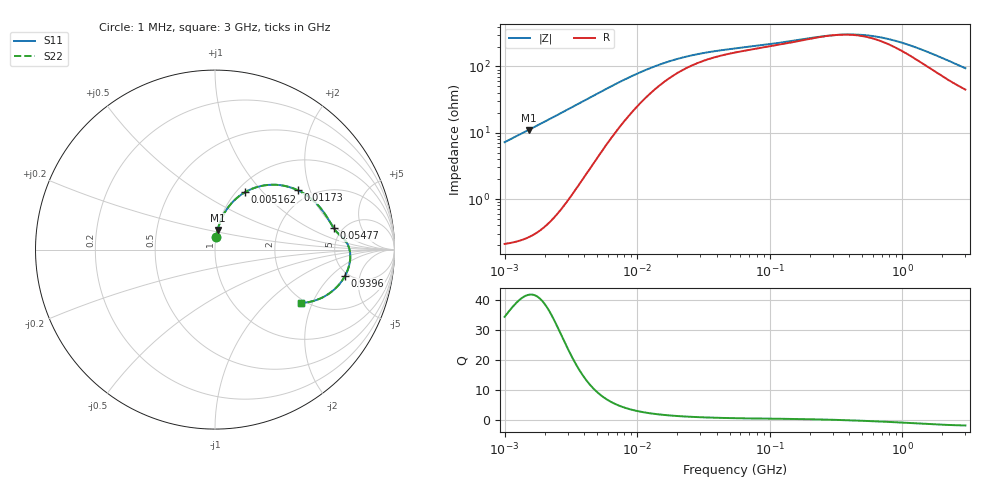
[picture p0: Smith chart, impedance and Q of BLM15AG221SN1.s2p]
! BLM15AG221SN1
# Hz S RI R 50
!Freq.(Hz) S11(Real) S11(Imag) S21(Real) S21(Imag) S12(Real) S12(Imag) S22(Real) S22(Imag)
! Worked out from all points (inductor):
!   401 points, 1 MHz to 3 GHz, reference 50 ohm
!   read as one part in series: L = 1.15 uH near 1.041 MHz
!   highest Q = 41.6 at 1.522 MHz (marker M1), where L = 1.16 uH
!   self-resonance near 321.7 MHz
!   S11 on the Smith chart (normalised r, x): 1 MHz: 1.00, +0.14; 5.162 MHz: 1.09, +0.80; 11.73 MHz: 1.69, +1.65; 54.77 MHz: 4.25, +1.85; 939.6 MHz: 4.65, -3.01; 3 GHz: 1.90, -1.65
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1000000  0.00723 0.0714  0.9928 -0.0714  0.9928 -0.0714  0.00723 0.0714
1522470  0.0146 0.1087  0.9854 -0.1087  0.9854 -0.1087  0.0146 0.1087
2561897  0.0405 0.1813  0.9595 -0.1813  0.9595 -0.1813  0.0405 0.1813
3823119  0.0927 0.2592  0.9073 -0.2592  0.9073 -0.2592  0.0927 0.2592
5161903  0.1659 0.3189  0.8341 -0.3189  0.8341 -0.3189  0.1659 0.3189
6433254  0.24 0.3502  0.76 -0.3502  0.76 -0.3502  0.24 0.3502
7703107  0.3085 0.3612  0.6915 -0.3612  0.6915 -0.3612  0.3085 0.3612
9410094  0.3848 0.3556  0.6152 -0.3556  0.6152 -0.3556  0.3848 0.3556
1.172775e7  0.4598 0.3314  0.5402 -0.3314  0.5402 -0.3314  0.4598 0.3314
1.461624e7  0.5199 0.296  0.4801 -0.296  0.4801 -0.296  0.5199 0.296
1.896016e7  0.5716 0.2501  0.4284 -0.2501  0.4284 -0.2501  0.5716 0.2501
2.509235e7  0.6085 0.2044  0.3915 -0.2044  0.3915 -0.2044  0.6085 0.2044
5.477226e7  0.6614 0.1196  0.3386 -0.1196  0.3386 -0.1196  0.6614 0.1196
2.094008e8  0.7326 0.0403  0.2674 -0.0403  0.2674 -0.0403  0.7326 0.0403
3.124888e8  0.7488 0.00307  0.2512 -0.00307  0.2512 -0.00307  0.7488 0.00307
4.304467e8  0.7538 -0.0334  0.2462 0.0334  0.2462 0.0334  0.7538 -0.0334
5.81181e8  0.7507 -0.0728  0.2493 0.0728  0.2493 0.0728  0.7507 -0.0728
8.005644e8  0.7366 -0.1207  0.2634 0.1207  0.2634 0.1207  0.7366 -0.1207
9.395906e8  0.7242 -0.1467  0.2758 0.1467  0.2758 0.1467  0.7242 -0.1467
1.613037e9  0.6457 -0.2378  0.3543 0.2378  0.3543 0.2378  0.6457 -0.2378
2.266846e9  0.5622 -0.2819  0.4378 0.2819  0.4378 0.2819  0.5622 -0.2819
3e9  0.4794 -0.2972  0.5206 0.2972  0.5206 0.2972  0.4794 -0.2972
